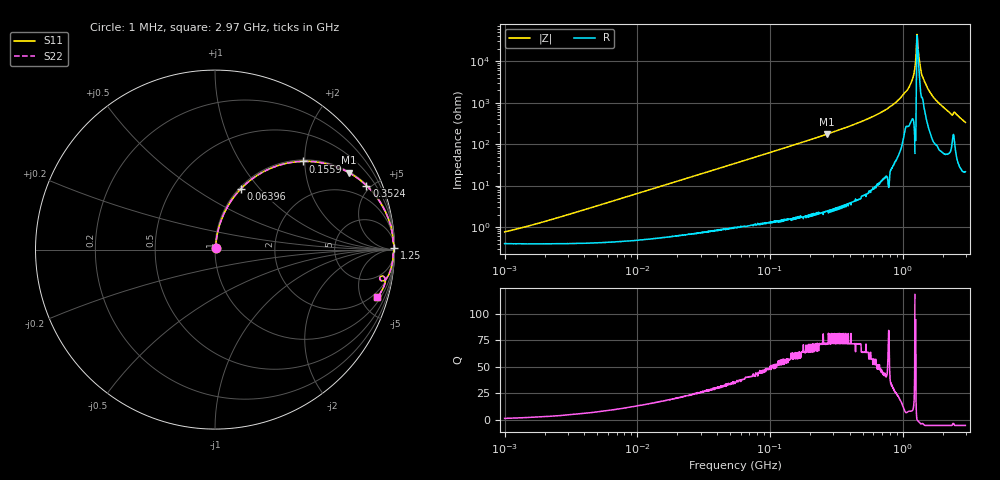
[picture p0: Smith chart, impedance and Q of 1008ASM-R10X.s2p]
!s-Parameter Generated by FASTRON Sdn. Bhd.
!FASTRON P/N : 1008ASM-R10X
!Keysight Technologies: E4991B_MY54100416_A.01.15
!Date: Mon Nov 20 15:57:41 2023
!Version  :Rev00  Wed Nov 22 15:11:40 2023
!Data & Calibration Information:
!Freq  S11  S21  S12  S22
!PortZ  Port1:50+j0  Port2:50+j0
!When reading reference impedance value at option line is always used.
! Remarks : This data is being provided solely for informational purposes.
# Hz S dB R 50
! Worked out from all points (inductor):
!   1599 points, 1 MHz to 2.97 GHz, reference 50 ohm
!   read as one part in series: L = 103 nH near 1.823 MHz
!   highest Q = 72.4 at 267.6 MHz (marker M1), where L = 103 nH
!   self-resonance near 1.288 GHz
!   S11 on the Smith chart (normalised r, x): 1 MHz: 1.01, +0.01; 63.96 MHz: 1.02, +0.80; 155.9 MHz: 1.03, +1.97; 352.4 MHz: 1.07, +4.71; 1.25 GHz: open; 2.97 GHz: 1.43, -6.64
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1000000  -42.40 58.1  -0.03 -0.4  -0.03 -0.4  -42.40 58.1
3804036  -32.10 79.3  -0.04 -1.4  -0.04 -1.4  -32.10 79.3
1.439846e7  -20.80 81.4  -0.08 -5.2  -0.08 -5.2  -20.80 81.4
5.477226e7  -9.82 69.6  -0.56 -18.8  -0.56 -18.8  -9.82 69.6
6.396315e7  -8.65 66.8  -0.73 -21.7  -0.73 -21.7  -8.65 66.8
1.558689e8  -3.16 45.0  -3.01 -44.0  -3.01 -44.0  -3.16 45.0
2.073156e8  -2.03 36.9  -4.44 -52.3  -4.44 -52.3  -2.03 36.9
2.675872e8  -1.30 29.8  -6.06 -59.4  -6.06 -59.4  -1.30 29.8
3.523638e8  -0.77 22.9  -8.18 -66.3  -8.18 -66.3  -0.77 22.9
7.846996e8  -0.09 7.5  -17.70 -81.8  -17.70 -81.8  -0.09 7.5
9.395906e8  -0.06 4.7  -21.70 -82.5  -21.70 -82.5  -0.06 4.7
1.11944e9  -0.05 2.4  -27.60 -80.9  -27.60 -80.9  -0.05 2.4
1.200675e9  -0.02 1.4  -32.50 -83.3  -32.50 -83.3  -0.02 1.4
1.249715e9  0.00 0.6  -39.60 -89.8  -39.60 -89.8  0.00 0.6
1.281378e9  -0.02 0.1  -52.90 -38.8  -52.90 -38.8  -0.02 0.1
1.307284e9  -0.03 -0.2  -46.00 44.1  -46.00 44.1  -0.03 -0.2
1.367504e9  -0.04 -0.9  -36.10 73.6  -36.10 73.6  -0.04 -0.9
1.423359e9  -0.06 -1.4  -32.10 72.3  -32.10 72.3  -0.06 -1.4
1.712864e9  -0.08 -4.2  -22.60 81.0  -22.60 81.0  -0.08 -4.2
2.289646e9  -0.32 -10.0  -15.10 73.1  -15.10 73.1  -0.32 -10.0
2.492946e9  -0.34 -9.8  -15.30 72.4  -15.30 72.4  -0.34 -9.8
2.970126e9  -0.53 -16.4  -11.00 69.9  -11.00 69.9  -0.53 -16.4
